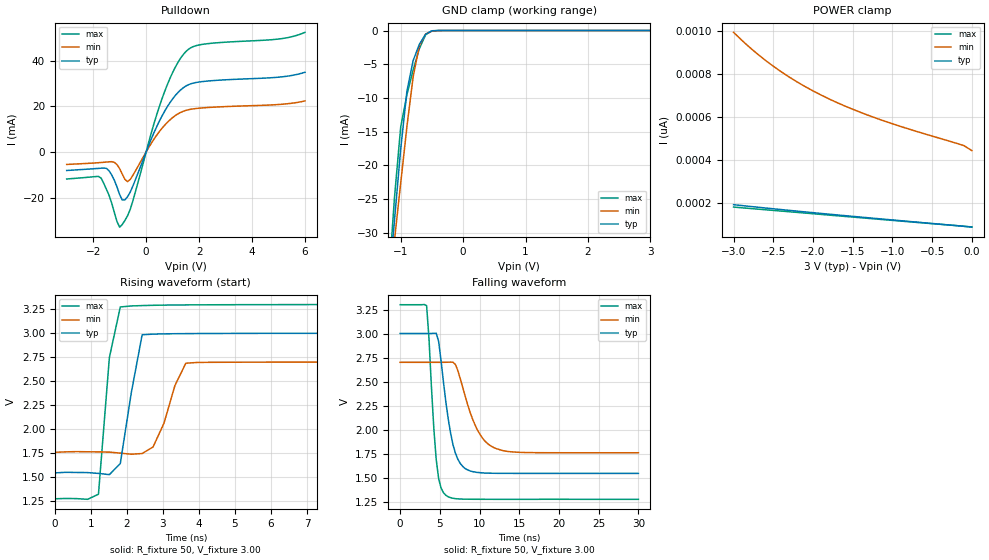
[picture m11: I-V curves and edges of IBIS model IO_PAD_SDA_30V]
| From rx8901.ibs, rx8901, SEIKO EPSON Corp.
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[Model]   IO_PAD_SDA_30V
Model_type I/O_open_drain
Enable Active-High
Polarity Non-Inverting
Vinh=2.10
Vinl=0.90
Vref=3.30
Vmeas=1.50
Rref=5000
C_comp   2.5p   2.0p   3.0p
[Temperature Range] 25   105   -40
[Voltage Range]   3.00   2.70   3.30
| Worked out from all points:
|   slope of the pulldown table from 0 to 0.45 V, typ, clamps not added: 36.6 ohm
|   GND clamp passes 1 mA (typ) near -0.63 V on its own axis
|   falling waveform, R_fixture 50, V_fixture 3.00: 20-80 % time 1.52ns typ, 2.45ns min, 890ps max; typ from 3 V to 1.54 V
|   rising waveform, R_fixture 50, V_fixture 3.00: 20-80 % time 389ps typ, 519ps min, 312ps max; typ from 1.54 V to 3 V
[Pulldown]
-3V       -8.089mA   -5.438mA   -11.81mA
-1.7V     -7.088mA   -4.591mA   -11.42mA
-1.4V     -8.196mA   -4.289mA   -18.94mA
-1V       -18.62mA   -7.291mA   -32.89mA
-800mV    -20.97mA   -12.01mA   -29.93mA
-600mV    -17.54mA   -12.01mA   -25.1mA
600mV     15.77mA    10.38mA    23.3mA
1.1V      24.7mA     15.93mA    37.08mA
1.5V      28.87mA    18.22mA    43.94mA
2.1V      30.79mA    19.28mA    47.07mA
5V        32.75mA    20.79mA    49.46mA
6V        34.91mA    22.36mA    52.39mA
[GND Clamp]
-3V       -252mA     -210.8mA   -302.4mA
-1.2V     -38.9mA    -39.62mA   -38.2mA
-1.1V     -28.19mA   -31.12mA   -24.82mA
-1V       -17.59mA   -22.65mA   -14.32mA
-900mV    -8.971mA   -14.23mA   -9.513mA
-800mV    -4.445mA   -6.839mA   -5.831mA
-700mV    -2.032mA   -2.214mA   -2.664mA
-600mV    -545.2uA   -526uA     -623.9uA
-500mV    -56.87uA   -82.5uA    -37.95uA
-400mV    -3.146uA   -8.827uA   -817.9nA
3V        88.06pA    490.1pA    79.4pA
[POWER Clamp]
-3V       192.6pA    994.4pA    181.4pA
-2.8V     184.8pA    925.3pA    175.2pA
-2.7V     181pA      893.9pA    172.1pA
-2.5V     173.5pA    836.8pA    165.9pA
-2.2V     162.6pA    763.7pA    156.6pA
-1.9V     152pA      703pA      147.4pA
-1.6V     141.6pA    651.8pA    138.1pA
-1.3V     131.5pA    607.8pA    128.8pA
-800mV    114.9pA    545.3pA    113.4pA
-100mV    91.86pA    467.4pA    92.29pA
0V        88.06pA    444.2pA    89.13pA
[Falling Waveform]
R_fixture=50
V_fixture=3.00
V_fixture_min=2.70
V_fixture_max=3.30
0s        3V         2.7V       3.3V
3.333ns   3V         2.7V       3.291V
4.545ns   3.003V     2.7V       1.685V
5.152ns   2.717V     2.7V       1.391V
5.758ns   2.287V     2.701V     1.315V
6.667ns   1.838V     2.7V       1.283V
7.576ns   1.647V     2.529V     1.276V
9.697ns   1.553V     2V         1.273V
11.82ns   1.544V     1.81V      1.273V
30ns      1.543V     1.758V     1.273V
[Rising Waveform]
R_fixture=50
V_fixture=3.00
V_fixture_min=2.70
V_fixture_max=3.30
0s        1.543V     1.758V     1.273V
1.212ns   1.537V     1.762V     1.32V
1.515ns   1.525V     1.76V      2.746V
1.818ns   1.641V     1.749V     3.274V
2.121ns   2.375V     1.738V     3.285V
2.424ns   2.984V     1.745V     3.289V
2.727ns   2.991V     1.813V     3.292V
3.333ns   2.995V     2.454V     3.295V
3.636ns   2.996V     2.687V     3.296V
30ns      3V         2.7V       3.3V
[Ramp]
R_load=50
dV/dt_r   8.743E-1/2.897E-10   5.653E-1/4.650E-10   1.216E+0/1.935E-10
dV/dt_f   8.743E-1/1.516E-9   5.653E-1/2.453E-9   1.216E+0/8.875E-10
|[End   IO_PAD_SDA_30V
